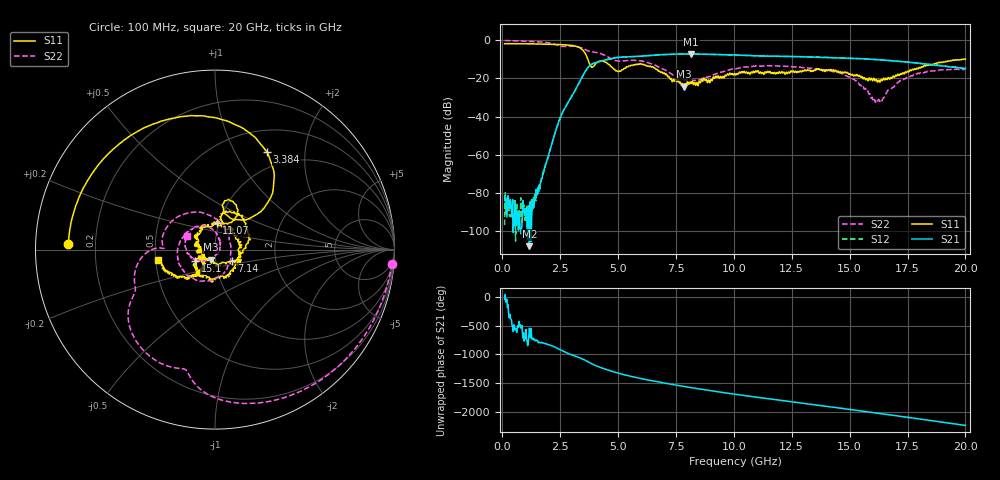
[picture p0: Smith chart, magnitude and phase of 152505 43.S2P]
!  2-Port S-parameters saved by WinCal
! VAR MeasName=S-Parameters (CALIBRATED_DATA) read from VNA (N5230C)
! VAR MeasDate=4/10/2015 9:32:46 AM
! VAR NAME=152505 43
! VAR FILENAME=152505 43.S2P
! VAR DATE=4/10/2015 9:32:46 AM
! VAR PHYS_PORTS=1,2
# Hz S DB R 50
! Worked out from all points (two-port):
!   801 points, 100 MHz to 20 GHz, reference 50 ohm
!   highest |S21| = -7.19 dB at 8.159 GHz (marker M1); lowest = -107.9 dB at 1.17 GHz (marker M2)
!   |S21| within 3 dB of the highest: 4.468 GHz to 16.22 GHz (11.75 GHz wide, 114 % of centre)
!   lowest |S11| = -24.2 dB at 7.836 GHz (marker M3), VSWR 1.13, Z = 47.4 - j5.42 ohm
!   |S11| at or under -10 dB: 3.699 GHz to 19.85 GHz (16.15 GHz wide, 137 % of centre); 19.89688 GHz to 19.9263 GHz (29.42 MHz wide, 0.148 % of centre)
!   |S22| runs from -32.4 to -0.1 dB; largest |S21 - S12| = 0.0069
!   S11 on the Smith chart (normalised r, x): 100 MHz: 0.10, +0.02; 3.384 GHz: 0.77, +1.36; 7.14 GHz: 1.19, -0.15; 11.07 GHz: 0.98, +0.30; 15.1 GHz: 0.79, -0.10; 20 GHz: 0.52, -0.07
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1e8  -1.75 177.6  -82.20 -37.8  -96.85 159.4  -0.08 -4.6
1.169625e9  -1.86 151.7  -107.87 178.1  -89.22 46.7  -0.53 -47.3
1.5925e9  -1.92 140.9  -75.90 -64.5  -75.87 -58.2  -0.82 -65.1
2.488e9  -2.20 112.6  -41.00 164.9  -41.01 164.6  -3.02 -102.1
3.3835e9  -4.20 62.1  -20.74 14.2  -20.75 14.6  -3.82 -137.2
3.43325e9  -4.66 58.2  -19.59 5.8  -19.58 6.1  -4.02 -139.9
3.856125e9  -14.16 59.5  -12.55 -82.4  -12.58 -82.2  -6.05 -152.9
4.52775e9  -11.93 59.4  -10.01 171.6  -10.03 171.7  -8.49 -178.1
5.32375e9  -14.54 80.0  -8.72 78.5  -8.71 78.7  -10.70 175.4
6.741625e9  -16.19 -1.5  -7.64 -41.0  -7.64 -41.1  -13.90 102.6
7.139625e9  -19.02 -34.6  -7.40 -70.8  -7.39 -70.6  -16.33 78.0
7.836125e9  -24.22 -112.2  -7.22 -120.2  -7.19 -120.0  -20.67 29.5
8.1595e9  -22.63 -146.9  -7.19 -141.6  -7.18 -141.6  -21.03 6.8
1.005e10  -17.49 138.5  -7.69 103.4  -7.75 103.1  -14.94 -103.3
1.106988e10  -16.52 86.1  -8.15 47.5  -8.14 47.4  -13.48 -143.3
1.221412e10  -17.84 -1.7  -8.45 -12.9  -8.45 -13.1  -13.60 -179.7
1.338325e10  -15.87 -80.8  -8.80 -75.1  -8.72 -74.7  -14.72 149.5
1.509962e10  -17.85 -149.9  -9.51 -166.7  -9.42 -166.8  -19.91 89.1
1.61195e10  -21.09 -143.1  -10.09 136.8  -10.08 136.6  -32.40 -11.7
1.669162e10  -19.63 -124.2  -10.58 105.1  -10.58 104.5  -25.97 -101.8
1.828362e10  -13.42 -133.8  -12.43 16.0  -12.37 16.4  -16.68 -168.3
2e10  -9.88 -169.1  -14.80 -82.1  -14.79 -82.0  -15.27 153.9
